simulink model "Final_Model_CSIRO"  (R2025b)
settings: Solver=ode23tb  StartTime=0.0  StopTime=50  RelTol=1e-3
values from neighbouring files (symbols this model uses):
  C_4 = 0.1670*C_b    (= 1.00487241952e-06)    [VSM_CSIRO.m]    (also in VSM.m)
  C_6 = 0.2835*C_b    (= 1.70587623314e-06)    [VSM_CSIRO.m]    (also in VSM.m)
  C_8 = 0.2275*C_b    (= 1.36891302659e-06)    [VSM_CSIRO.m]    (also in VSM.m)
  C_dc = 0.008*(n)    (= 1.6)    [VSM_CSIRO.m]    (also in VSM.m)
  C_f = n*300*10^-6    (= 0.06)    [VSM_CSIRO.m]    (also in VSM.m)
  D_p = (1/(m_p*w_b))    (= 101321.183642)    [VSM_CSIRO.m]    (also in VSM.m)
  droop_percentage = 1    [VSM_CSIRO.m]    (also in VSM.m = 5)
  i_ll = -1.15*(S_b/Vdc_n)-i_loss_dc    [VSM_CSIRO.m]    (also in VSM.m)
  i_ul = 1.15*(S_b/Vdc_n)+i_loss_dc    [VSM_CSIRO.m]    (also in VSM.m)
  J = D_p*tau_f    (= 2026.42367285)    [VSM_CSIRO.m]    (also in VSM.m)
  k_dc = eta_1/(Vdc_n*m_p)    [VSM_CSIRO.m]    (also in VSM.m)
  K_p = (1/Vdc_n)    [VSM_CSIRO.m]    (also in VSM.m)
  K_r = 1/R_dc    [VSM_CSIRO.m]    (also in VSM.m)
  Kff_i = 1    [VSM_CSIRO.m]    (also in VSM.m)
  Kff_v = 1    [VSM_CSIRO.m]    (also in VSM.m)
  Ki_i = (1/n)*1.19    (= 0.00595)    [VSM_CSIRO.m]    (also in VSM.m)
  Ki_v = (n)*1.161022    (= 232.2044)    [VSM_CSIRO.m]    (also in VSM.m)
  ki_v_ac = 4*5.2500e-04    (= 0.0021)    [VSM_CSIRO.m]    (also in VSM.m)
  Kp_i = 0.738891    [VSM_CSIRO.m]    (also in VSM.m)
  Kp_v = 0.52    [VSM_CSIRO.m]    (also in VSM.m)
  kp_v_ac = 0.001    [VSM_CSIRO.m]    (also in VSM.m)
  L1_pu = 1*0.0186/m    (= 0.000186)    [VSM_CSIRO.m]    (also in VSM.m)
  L_45 = L_lines(2)    [VSM_CSIRO.m]    (also in VSM.m)
  L_56 = L_lines(3)    [VSM_CSIRO.m]    (also in VSM.m)
  L_67 = L_lines(5)    [VSM_CSIRO.m]    (also in VSM.m)
  L_78 = L_lines(6)    [VSM_CSIRO.m]    (also in VSM.m)
  L_89 = L_lines(8)    [VSM_CSIRO.m]    (also in VSM.m)
  L_94 = L_lines(9)    [VSM_CSIRO.m]    (also in VSM.m)
  L_f = (1/n)*200*10^-6    (= 1e-06)    [VSM_CSIRO.m]    (also in VSM.m)
  n = 200    [VSM_CSIRO.m]    (also in VSM.m)
  pl = S_b*ps    (= 75000000)    [VSM_CSIRO.m]    (also in VSM.m)
  ps = base/3    (= 0.75)    [VSM_CSIRO.m]    (also in VSM.m)
  R1_pu = 1*0.00734/m    (= 7.34e-05)    [VSM_CSIRO.m]    (also in VSM.m)
  R_45 = R_lines(2)    [VSM_CSIRO.m]    (also in VSM.m)
  R_56 = R_lines(3)    [VSM_CSIRO.m]    (also in VSM.m)
  R_67 = R_lines(5)    [VSM_CSIRO.m]    (also in VSM.m)
  R_78 = R_lines(6)    [VSM_CSIRO.m]    (also in VSM.m)
  R_89 = R_lines(8)    [VSM_CSIRO.m]    (also in VSM.m)
  R_94 = R_lines(9)    [VSM_CSIRO.m]    (also in VSM.m)
  R_dc = (Vdc_n/(0.05*(S_b)/Vdc_n))    [VSM_CSIRO.m]    (also in VSM.m)
  R_f = 0.001/n    (= 5e-06)    [VSM_CSIRO.m]    (also in VSM.m)
  S_b = 100*(10^6)    (= 100000000)    [VSM_CSIRO.m]    (also in VSM.m)
  S_bt = S_b    (= 100000000)    [VSM_CSIRO.m]    (also in VSM.m)
  T_en = T_load-0.5    (= 44.5)    [VSM_CSIRO.m]    (also in VSM.m = 24.5)
  t_l = 2    [VSM_CSIRO.m]
  tau_dc = 0.05    [VSM_CSIRO.m]    (also in VSM.m)
  tau_g = 5    [VSM_CSIRO.m]    (also in VSM.m)
  V1_rms = 1000    [VSM_CSIRO.m]    (also in VSM.m)
  V2_rms = 13800    [VSM_CSIRO.m]    (also in VSM.m)
  V_m = sqrt(2/3)*V1_rms    [VSM_CSIRO.m]    (also in VSM.m)
  Vdc_n = 3*V_m    [VSM_CSIRO.m]    (also in VSM.m)
  w_b = 2*pi*f_b    (= 314.159265359)    [VSM_CSIRO.m]    (also in VSM.m)
  w_f = 2*pi*5    (= 31.4159265359)    [VSM_CSIRO.m]    (also in VSM.m)
undefined symbols (not defined in the file or in its folder): D1, Delta, DiscIntNeverNeededParam, i_dc
libraries: spsSeriesRLCBranchLib x142, spsThreePhaseVIMeasurementLib x69, slpidlib x44, spsabctodq0Lib x44, spsVoltageMeasurementLib x28, spsGroundLib x23, spsThreePhaseBreakerLib x23, spsThreePhaseParallelRLCLoadLib x21, spsdq0toabcLib x16, spsUniversalBridgeLib x16, spsPowerPositiveSequenceLib x14, spsDCVoltageSourceLib x14
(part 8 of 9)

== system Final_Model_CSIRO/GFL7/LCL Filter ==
  Cf : spsSeriesRLCBranchLib/Series RLC Branch  LConnTagsString=__new0  RConnTagsString=__new0  BranchType=RC  Resistance=200  Inductance=0.0058  SetiL0=off  InitialCurrent=0  Capacitance=50e-6  Setx0=off  InitialVoltage=0  Measurements=None
  Cf1 : spsSeriesRLCBranchLib/Series RLC Branch  LConnTagsString=__new0  RConnTagsString=__new0  BranchType=RC  Resistance=200  Inductance=0.0058  SetiL0=off  InitialCurrent=0  Capacitance=50e-6  Setx0=off  InitialVoltage=0  Measurements=None
  Cf2 : spsSeriesRLCBranchLib/Series RLC Branch  LConnTagsString=__new0  RConnTagsString=__new0  BranchType=RC  Resistance=200  Inductance=0.0058  SetiL0=off  InitialCurrent=0  Capacitance=50e-6  Setx0=off  InitialVoltage=0  Measurements=None
  Ground : spsGroundLib/Ground  LConnTagsString=a
  Lg : spsSeriesRLCBranchLib/Series RLC Branch  LConnTagsString=__new0  RConnTagsString=__new0  BranchType=L  Resistance=0.2  Inductance=5e-6  SetiL0=off  InitialCurrent=0  Capacitance=1e-6  Setx0=off  InitialVoltage=0  Measurements=None
  Linv : spsSeriesRLCBranchLib/Series RLC Branch  LConnTagsString=__new0  RConnTagsString=__new0  BranchType=RL  Resistance=1e-3  Inductance=0.003e-3  SetiL0=off  InitialCurrent=0  Capacitance=1e-6  Setx0=off  InitialVoltage=0  Measurements=None
  Series RLC Branch1 : spsSeriesRLCBranchLib/Series RLC Branch  LConnTagsString=__new0  RConnTagsString=__new0  BranchType=RL  Resistance=1e-3  Inductance=0.003e-3  SetiL0=off  InitialCurrent=0  Capacitance=1e-6  Setx0=off  InitialVoltage=0  Measurements=None
  Series RLC Branch2 : spsSeriesRLCBranchLib/Series RLC Branch  LConnTagsString=__new0  RConnTagsString=__new0  BranchType=RL  Resistance=1e-3  Inductance=0.003e-3  SetiL0=off  InitialCurrent=0  Capacitance=1e-6  Setx0=off  InitialVoltage=0  Measurements=None
  Series RLC Branch3 : spsSeriesRLCBranchLib/Series RLC Branch  LConnTagsString=__new0  RConnTagsString=__new0  BranchType=L  Resistance=0.2  Inductance=5e-6  SetiL0=off  InitialCurrent=0  Capacitance=1e-6  Setx0=off  InitialVoltage=0  Measurements=None
  Series RLC Branch4 : spsSeriesRLCBranchLib/Series RLC Branch  LConnTagsString=__new0  RConnTagsString=__new0  BranchType=L  Resistance=0.2  Inductance=5e-6  SetiL0=off  InitialCurrent=0  Capacitance=1e-6  Setx0=off  InitialVoltage=0  Measurements=None
  Three-Phase V-I Measurement : spsThreePhaseVIMeasurementLib/Three-Phase V-I Measurement  VoltageMeasurement=phase-to-phase  SetLabelV=on  LabelV=Vabc_B2_8  Vpu=off  VpuLL=off  CurrentMeasurement=no  SetLabelI=off  LabelI=Iabc  Ipu=off  Pbase=100e6  Vbase=500e3  OutputType=Complex  PhasorSimulation=off  PSBequivalent=0
  A : PMIOPort  Side=Left
  a : PMIOPort  Port=2  Side=Right
  B : PMIOPort  Port=3  Side=Left
  b : PMIOPort  Port=4  Side=Right
  C : PMIOPort  Port=5  Side=Left
  c : PMIOPort  Port=6  Side=Right
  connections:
  A/RConn1 -- Linv/LConn1
  B/RConn1 -- Series RLC Branch1/LConn1
  C/RConn1 -- Series RLC Branch2/LConn1
  Lg/LConn1 -- Three-Phase V-I Measurement/LConn1 -- Linv/RConn1
  Series RLC Branch4/LConn1 -- Three-Phase V-I Measurement/LConn3 -- Series RLC Branch2/RConn1
  Series RLC Branch3/LConn1 -- Three-Phase V-I Measurement/LConn2 -- Series RLC Branch1/RConn1
  Cf1/LConn1 -- Ground/LConn1 -- Cf/LConn1 -- Cf2/LConn1
  Cf/RConn1 -- Three-Phase V-I Measurement/RConn1
  Cf1/RConn1 -- Three-Phase V-I Measurement/RConn2
  Cf2/RConn1 -- Three-Phase V-I Measurement/RConn3
  Lg/RConn1 -- a/RConn1
  Series RLC Branch3/RConn1 -- b/RConn1
  Series RLC Branch4/RConn1 -- c/RConn1

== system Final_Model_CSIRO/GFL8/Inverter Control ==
  note: PLL
  Vabc_B3 : Inport
  Iabc_B3 : Inport  Port=2
  Idref : Inport  Port=3
  Iqref : Inport  Port=4
  Clock : Clock
  Constant : Constant  Value=0  SampleTime=-1
  Constant1 : Constant  Value=0  SampleTime=-1
  Constant3 : Constant  Value=314.159  SampleTime=-1
  Constant4 : Constant  Value=0
  Demux : Demux  Outputs=3
  Demux1 : Demux  Outputs=3
  Discrete-Time Integrator : DiscreteIntegrator  SampleTime=-1  ICPrevOutput=DiscIntNeverNeededParam  ICPrevScaledInput=DiscIntNeverNeededParam
  Gain : Gain  Gain=2/1800
  Memory : Memory
  Mux : Mux  Inputs=3
  PID Controller : slpidlib/PID Controller  Controller=PI  Form=Parallel  TimeDomain=Discrete-time  UseExternalTs=off  SampleTime=-1  IntegratorMethod=Forward Euler  FilterMethod=Forward Euler  ControllerParametersSource=internal  P=0.02  I=50  UseKiTs=off  D=0  UseExternalDerivativeSource=off  N=100  UseFilter=on  TunerSelectOption=Transfer Function Based (PID Tuner App)  InitialConditionSource=internal  InitialConditionForIntegrator=0  InitialConditionForFilter=0  DifferentiatorICPrevScaledInput=0  ExternalReset=none  TrackingMode=off  Kt=1  LimitOutput=off  SatLimitsSource=internal  UpperSaturationLimit=inf  LowerSaturationLimit=-inf  LinearizeAsGain=on  AntiWindupMode=none  Kb=1  LimitIntegrator=off  UpperIntegratorSaturationLimit=inf  LowerIntegratorSaturationLimit=-inf  POutMin=[]  POutMax=[]  IOutMin=[]  IOutMax=[]  DOutMin=[]  DOutMax=[]  NOutMin=[]  NOutMax=[]  SumOutMin=[]  SumOutMax=[]  SaturationOutMin=[]  SaturationOutMax=[]  PParamMin=[]  PParamMax=[]  IParamMin=[]  IParamMax=[]  DParamMin=[]  DParamMax=[]  NParamMin=[]  NParamMax=[]  KbParamMin=[]  KbParamMax=[]  KtParamMin=[]  KtParamMax=[]  KbOutMin=[]  KbOutMax=[]  KtOutMin=[]  KtOutMax=[]  IntegratorOutMin=[]  IntegratorOutMax=[]  FilterOutMin=[]  FilterOutMax=[]  SumI1OutMin=[]  SumI1OutMax=[]  SumI2OutMin=[]  SumI2OutMax=[]  SumI3OutMin=[]  SumI3OutMax=[]  SumI4OutMin=[]  SumI4OutMax=[]  SumDOutMin=[]  SumDOutMax=[]  DifferentiatorOutMin=[]  DifferentiatorOutMax=[]  FilterDiffOutCoefMin=[]  FilterDiffOutCoefMax=[]  ReciprocalOutMin=[]  ReciprocalOutMax=[]  SumDenOutMin=[]  SumDenOutMax=[]  SumNumOutMin=[]  SumNumOutMax=[]  DivideOutMin=[]  DivideOutMax=[]  UdiffTsProdOutMin=[]  UdiffTsProdOutMax=[]  NTsProdOutMin=[]  NTsProdOutMax=[]  UintegralTsProdOutMin=[]  UintegralTsProdOutMax=[]  UngainTsProdOutMin=[]  UngainTsProdOutMax=[]  ClampingZeroOutDataTypeStr=Inherit: Inherit via back propagation  ClampingZeroOutMin=[]  ClampingZeroOutMax=[]  FilterDenConstantOutDataTypeStr=Inherit: Inherit via back propagation  FilterDenConstantOutMin=[]  FilterDenConstantOutMax=[]  PCopyOutDataTypeStr=Inherit: Inherit via back propagation  PCopyOutMin=[]  PCopyOutMax=[]  NCopyOutDataTypeStr=Inherit: Inherit via back propagation  NCopyOutMin=[]  NCopyOutMax=[]  IntegratorContinuousStateAttributes=''  IntegratorStateMustResolveToSignalObject=off  IntegratorRTWStateStorageClass=Auto  FilterContinuousStateAttributes=''  FilterStateMustResolveToSignalObject=off  FilterRTWStateStorageClass=Auto  ParallelPVariant=InternalParameters  IdealPVariant=Disabled  IVariant=InternalParameters  DVariant=Disabled  IntegratorVariant=Discrete  SatVariant=Disabled  AWVariant=Passthrough  PCopyVariant=Disabled  TRVariant=Disabled  FdbkBlocksVariant=Forward  IdealPFdbkVariant=Disabled  SatFdbkVariant=Disabled  DerivativeFilterVariant=Disabled  NVariant=Disabled  NCopyVariant=Disabled_SignalSpec  FilterICVariant=Disabled  IntegratorICVariant=InternalICs  ExternalResetVariant=Disabled  TRSumVariant=Passthrough  SumFdbkVariant=Disabled  SumVariant=Sum_PI  TsampFilterVariant=InternalTs  TsampNgainVariant=Passthrough  TsampIntegralVariant=Disabled_SignalSpec  ExternalSaturationOutDataTypeStr=Inherit: Same as second input  DerivativeSourceVariant=Disabled  PreIntVariant=InternalPreInt
  PID Controller1 : slpidlib/PID Controller  Controller=PI  Form=Parallel  TimeDomain=Discrete-time  UseExternalTs=off  SampleTime=-1  IntegratorMethod=Forward Euler  FilterMethod=Forward Euler  ControllerParametersSource=internal  P=0.1  I=10000/200  UseKiTs=off  D=0  UseExternalDerivativeSource=off  N=100  UseFilter=on  TunerSelectOption=Transfer Function Based (PID Tuner App)  InitialConditionSource=internal  InitialConditionForIntegrator=0  InitialConditionForFilter=0  DifferentiatorICPrevScaledInput=0  ExternalReset=none  TrackingMode=off  Kt=1  LimitOutput=on  SatLimitsSource=internal  UpperSaturationLimit=20e3  LowerSaturationLimit=-20e3  LinearizeAsGain=on  AntiWindupMode=none  Kb=1  LimitIntegrator=off  UpperIntegratorSaturationLimit=inf  LowerIntegratorSaturationLimit=-inf  POutMin=[]  POutMax=[]  IOutMin=[]  IOutMax=[]  DOutMin=[]  DOutMax=[]  NOutMin=[]  NOutMax=[]  SumOutMin=[]  SumOutMax=[]  SaturationOutMin=[]  SaturationOutMax=[]  PParamMin=[]  PParamMax=[]  IParamMin=[]  IParamMax=[]  DParamMin=[]  DParamMax=[]  NParamMin=[]  NParamMax=[]  KbParamMin=[]  KbParamMax=[]  KtParamMin=[]  KtParamMax=[]  KbOutMin=[]  KbOutMax=[]  KtOutMin=[]  KtOutMax=[]  IntegratorOutMin=[]  IntegratorOutMax=[]  FilterOutMin=[]  FilterOutMax=[]  SumI1OutMin=[]  SumI1OutMax=[]  SumI2OutMin=[]  SumI2OutMax=[]  SumI3OutMin=[]  SumI3OutMax=[]  SumI4OutMin=[]  SumI4OutMax=[]  SumDOutMin=[]  SumDOutMax=[]  DifferentiatorOutMin=[]  DifferentiatorOutMax=[]  FilterDiffOutCoefMin=[]  FilterDiffOutCoefMax=[]  ReciprocalOutMin=[]  ReciprocalOutMax=[]  SumDenOutMin=[]  SumDenOutMax=[]  SumNumOutMin=[]  SumNumOutMax=[]  DivideOutMin=[]  DivideOutMax=[]  UdiffTsProdOutMin=[]  UdiffTsProdOutMax=[]  NTsProdOutMin=[]  NTsProdOutMax=[]  UintegralTsProdOutMin=[]  UintegralTsProdOutMax=[]  UngainTsProdOutMin=[]  UngainTsProdOutMax=[]  ClampingZeroOutDataTypeStr=Inherit: Inherit via back propagation  ClampingZeroOutMin=[]  ClampingZeroOutMax=[]  FilterDenConstantOutDataTypeStr=Inherit: Inherit via back propagation  FilterDenConstantOutMin=[]  FilterDenConstantOutMax=[]  PCopyOutDataTypeStr=Inherit: Inherit via back propagation  PCopyOutMin=[]  PCopyOutMax=[]  NCopyOutDataTypeStr=Inherit: Inherit via back propagation  NCopyOutMin=[]  NCopyOutMax=[]  IntegratorContinuousStateAttributes=''  IntegratorStateMustResolveToSignalObject=off  IntegratorRTWStateStorageClass=Auto  FilterContinuousStateAttributes=''  FilterStateMustResolveToSignalObject=off  FilterRTWStateStorageClass=Auto  ParallelPVariant=InternalParameters  IdealPVariant=Disabled  IVariant=InternalParameters  DVariant=Disabled  IntegratorVariant=Discrete  SatVariant=Enabled  AWVariant=Passthrough  PCopyVariant=Disabled  TRVariant=Disabled  FdbkBlocksVariant=Forward  IdealPFdbkVariant=Disabled  SatFdbkVariant=Disabled  DerivativeFilterVariant=Disabled  NVariant=Disabled  NCopyVariant=Disabled_SignalSpec  FilterICVariant=Disabled  IntegratorICVariant=InternalICs  ExternalResetVariant=Disabled  TRSumVariant=Passthrough  SumFdbkVariant=Disabled  SumVariant=Sum_PI  TsampFilterVariant=InternalTs  TsampNgainVariant=Passthrough  TsampIntegralVariant=Disabled_SignalSpec  ExternalSaturationOutDataTypeStr=Inherit: Same as second input  DerivativeSourceVariant=Disabled  PreIntVariant=InternalPreInt
  PID Controller2 : slpidlib/PID Controller  Controller=PI  Form=Parallel  TimeDomain=Discrete-time  UseExternalTs=off  SampleTime=-1  IntegratorMethod=Forward Euler  FilterMethod=Forward Euler  ControllerParametersSource=internal  P=0.1  I=1000/2  UseKiTs=off  D=0  UseExternalDerivativeSource=off  N=100  UseFilter=on  TunerSelectOption=Transfer Function Based (PID Tuner App)  InitialConditionSource=internal  InitialConditionForIntegrator=0  InitialConditionForFilter=0  DifferentiatorICPrevScaledInput=0  ExternalReset=none  TrackingMode=off  Kt=1  LimitOutput=on  SatLimitsSource=internal  UpperSaturationLimit=20e3  LowerSaturationLimit=-20e3  LinearizeAsGain=on  AntiWindupMode=none  Kb=1  LimitIntegrator=off  UpperIntegratorSaturationLimit=inf  LowerIntegratorSaturationLimit=-inf  POutMin=[]  POutMax=[]  IOutMin=[]  IOutMax=[]  DOutMin=[]  DOutMax=[]  NOutMin=[]  NOutMax=[]  SumOutMin=[]  SumOutMax=[]  SaturationOutMin=[]  SaturationOutMax=[]  PParamMin=[]  PParamMax=[]  IParamMin=[]  IParamMax=[]  DParamMin=[]  DParamMax=[]  NParamMin=[]  NParamMax=[]  KbParamMin=[]  KbParamMax=[]  KtParamMin=[]  KtParamMax=[]  KbOutMin=[]  KbOutMax=[]  KtOutMin=[]  KtOutMax=[]  IntegratorOutMin=[]  IntegratorOutMax=[]  FilterOutMin=[]  FilterOutMax=[]  SumI1OutMin=[]  SumI1OutMax=[]  SumI2OutMin=[]  SumI2OutMax=[]  SumI3OutMin=[]  SumI3OutMax=[]  SumI4OutMin=[]  SumI4OutMax=[]  SumDOutMin=[]  SumDOutMax=[]  DifferentiatorOutMin=[]  DifferentiatorOutMax=[]  FilterDiffOutCoefMin=[]  FilterDiffOutCoefMax=[]  ReciprocalOutMin=[]  ReciprocalOutMax=[]  SumDenOutMin=[]  SumDenOutMax=[]  SumNumOutMin=[]  SumNumOutMax=[]  DivideOutMin=[]  DivideOutMax=[]  UdiffTsProdOutMin=[]  UdiffTsProdOutMax=[]  NTsProdOutMin=[]  NTsProdOutMax=[]  UintegralTsProdOutMin=[]  UintegralTsProdOutMax=[]  UngainTsProdOutMin=[]  UngainTsProdOutMax=[]  ClampingZeroOutDataTypeStr=Inherit: Inherit via back propagation  ClampingZeroOutMin=[]  ClampingZeroOutMax=[]  FilterDenConstantOutDataTypeStr=Inherit: Inherit via back propagation  FilterDenConstantOutMin=[]  FilterDenConstantOutMax=[]  PCopyOutDataTypeStr=Inherit: Inherit via back propagation  PCopyOutMin=[]  PCopyOutMax=[]  NCopyOutDataTypeStr=Inherit: Inherit via back propagation  NCopyOutMin=[]  NCopyOutMax=[]  IntegratorContinuousStateAttributes=''  IntegratorStateMustResolveToSignalObject=off  IntegratorRTWStateStorageClass=Auto  FilterContinuousStateAttributes=''  FilterStateMustResolveToSignalObject=off  FilterRTWStateStorageClass=Auto  ParallelPVariant=InternalParameters  IdealPVariant=Disabled  IVariant=InternalParameters  DVariant=Disabled  IntegratorVariant=Discrete  SatVariant=Enabled  AWVariant=Passthrough  PCopyVariant=Disabled  TRVariant=Disabled  FdbkBlocksVariant=Forward  IdealPFdbkVariant=Disabled  SatFdbkVariant=Disabled  DerivativeFilterVariant=Disabled  NVariant=Disabled  NCopyVariant=Disabled_SignalSpec  FilterICVariant=Disabled  IntegratorICVariant=InternalICs  ExternalResetVariant=Disabled  TRSumVariant=Passthrough  SumFdbkVariant=Disabled  SumVariant=Sum_PI  TsampFilterVariant=InternalTs  TsampNgainVariant=Passthrough  TsampIntegralVariant=Disabled_SignalSpec  ExternalSaturationOutDataTypeStr=Inherit: Same as second input  DerivativeSourceVariant=Disabled  PreIntVariant=InternalPreInt
  Saturation : Saturate  UpperLimit=1  LowerLimit=-1
  Scope : Scope  NumInputPorts=2
  Scope4 : Scope  NumInputPorts=2
  Sum : Sum  Inputs=|-+
  Sum1 : Sum  Inputs=|+-
  Sum2 : Sum  Inputs=|+-
  Sum3 : Sum  Inputs=|+-
  Sum{4..6,8} (4 alike) : Sum  Inputs=|++
  Switch : Switch  Criteria=u2 > Threshold  Threshold=10
  Terminator : Terminator
  Terminator1 : Terminator
  abc to dq0 : spsabctodq0Lib/abc to dq0  Alignment=90 degrees behind phase A axis
  abc to dq1 : spsabctodq0Lib/abc to dq0  Alignment=90 degrees behind phase A axis
  dq0 to abc : spsdq0toabcLib/dq0 to abc  Alignment=90 degrees behind phase A axis
  wL : Gain  Gain=0.314*0.003
  wL1 : Gain  Gain=0.314*0.003
  Pulses : Outport
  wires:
  abc to dq0/1 -> Demux/1
  Demux/3 -> Terminator/1
  Demux1/3 -> Terminator1/1
  abc to dq1/1 -> Demux1/1
  Iabc_B3/1 -> abc to dq1/1
  Constant/1 -> Sum/1
  Demux/2 -> [Vq]  "Vq"
  Sum/1 -> PID Controller/1
  PID Controller/1 -> Sum8/1
  [wt] -> abc to dq1/2, abc to dq0/2
  Demux1/1 -> [Id]  "Id"
  Demux1/2 -> [Iq]  "Iq"
  [Id] -> Scope/2, Sum1/2
  Iqref/1 -> Scope4/1, Sum2/1
  [Iq] -> Sum2/2, Scope4/2
  Sum1/1 -> PID Controller1/1
  Sum2/1 -> PID Controller2/1
  PID Controller1/1 -> Sum3/1
  PID Controller2/1 -> Sum4/1
  wL1/1 -> Sum4/2
  wL/1 -> Sum3/2
  Sum3/1 -> Sum5/1
  [Vd] -> Sum5/2
  Sum4/1 -> Sum6/1
  [Vq] -> Sum6/2
  Mux/1 -> dq0 to abc/1
  Sum5/1 -> Mux/1  "ud"
  Sum6/1 -> Mux/2  "uq"
  Constant1/1 -> Mux/3
  dq0 to abc/1 -> Gain/1
  Vabc_B3/1 -> abc to dq0/1
  Idref/1 -> Scope/1, Sum1/1
  [Id] -> wL1/1
  [Iq] -> wL/1
  Demux/1 -> [Vd]  "Vd"
  Gain/1 -> Saturation/1
  Memory/1 -> Pulses/1
  Discrete-Time Integrator/1 -> [wt]
  Saturation/1 -> Memory/1
  Constant3/1 -> Sum8/2
  Switch/1 -> Sum/2
  Constant4/1 -> Switch/3
  Clock/1 -> Switch/2
  [Vq] -> Switch/1
  [wt] -> dq0 to abc/2
  Sum8/1 -> Discrete-Time Integrator/1

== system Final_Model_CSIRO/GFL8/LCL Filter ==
  Cf : spsSeriesRLCBranchLib/Series RLC Branch  LConnTagsString=__new0  RConnTagsString=__new0  BranchType=RC  Resistance=200  Inductance=0.0058  SetiL0=off  InitialCurrent=0  Capacitance=50e-6  Setx0=off  InitialVoltage=0  Measurements=None
  Cf1 : spsSeriesRLCBranchLib/Series RLC Branch  LConnTagsString=__new0  RConnTagsString=__new0  BranchType=RC  Resistance=200  Inductance=0.0058  SetiL0=off  InitialCurrent=0  Capacitance=50e-6  Setx0=off  InitialVoltage=0  Measurements=None
  Cf2 : spsSeriesRLCBranchLib/Series RLC Branch  LConnTagsString=__new0  RConnTagsString=__new0  BranchType=RC  Resistance=200  Inductance=0.0058  SetiL0=off  InitialCurrent=0  Capacitance=50e-6  Setx0=off  InitialVoltage=0  Measurements=None
  Ground : spsGroundLib/Ground  LConnTagsString=a
  Lg : spsSeriesRLCBranchLib/Series RLC Branch  LConnTagsString=__new0  RConnTagsString=__new0  BranchType=L  Resistance=0.2  Inductance=5e-6  SetiL0=off  InitialCurrent=0  Capacitance=1e-6  Setx0=off  InitialVoltage=0  Measurements=None
  Linv : spsSeriesRLCBranchLib/Series RLC Branch  LConnTagsString=__new0  RConnTagsString=__new0  BranchType=RL  Resistance=1e-3  Inductance=0.003e-3  SetiL0=off  InitialCurrent=0  Capacitance=1e-6  Setx0=off  InitialVoltage=0  Measurements=None
  Series RLC Branch1 : spsSeriesRLCBranchLib/Series RLC Branch  LConnTagsString=__new0  RConnTagsString=__new0  BranchType=RL  Resistance=1e-3  Inductance=0.003e-3  SetiL0=off  InitialCurrent=0  Capacitance=1e-6  Setx0=off  InitialVoltage=0  Measurements=None
  Series RLC Branch2 : spsSeriesRLCBranchLib/Series RLC Branch  LConnTagsString=__new0  RConnTagsString=__new0  BranchType=RL  Resistance=1e-3  Inductance=0.003e-3  SetiL0=off  InitialCurrent=0  Capacitance=1e-6  Setx0=off  InitialVoltage=0  Measurements=None
  Series RLC Branch3 : spsSeriesRLCBranchLib/Series RLC Branch  LConnTagsString=__new0  RConnTagsString=__new0  BranchType=L  Resistance=0.2  Inductance=5e-6  SetiL0=off  InitialCurrent=0  Capacitance=1e-6  Setx0=off  InitialVoltage=0  Measurements=None
  Series RLC Branch4 : spsSeriesRLCBranchLib/Series RLC Branch  LConnTagsString=__new0  RConnTagsString=__new0  BranchType=L  Resistance=0.2  Inductance=5e-6  SetiL0=off  InitialCurrent=0  Capacitance=1e-6  Setx0=off  InitialVoltage=0  Measurements=None
  Three-Phase V-I Measurement : spsThreePhaseVIMeasurementLib/Three-Phase V-I Measurement  VoltageMeasurement=phase-to-phase  SetLabelV=on  LabelV=Vabc_B2_9  Vpu=off  VpuLL=off  CurrentMeasurement=no  SetLabelI=off  LabelI=Iabc  Ipu=off  Pbase=100e6  Vbase=500e3  OutputType=Complex  PhasorSimulation=off  PSBequivalent=0
  A : PMIOPort  Side=Left
  a : PMIOPort  Port=2  Side=Right
  B : PMIOPort  Port=3  Side=Left
  b : PMIOPort  Port=4  Side=Right
  C : PMIOPort  Port=5  Side=Left
  c : PMIOPort  Port=6  Side=Right
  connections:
  A/RConn1 -- Linv/LConn1
  B/RConn1 -- Series RLC Branch1/LConn1
  C/RConn1 -- Series RLC Branch2/LConn1
  Lg/LConn1 -- Three-Phase V-I Measurement/LConn1 -- Linv/RConn1
  Series RLC Branch4/LConn1 -- Three-Phase V-I Measurement/LConn3 -- Series RLC Branch2/RConn1
  Series RLC Branch3/LConn1 -- Three-Phase V-I Measurement/LConn2 -- Series RLC Branch1/RConn1
  Cf1/LConn1 -- Ground/LConn1 -- Cf/LConn1 -- Cf2/LConn1
  Cf/RConn1 -- Three-Phase V-I Measurement/RConn1
  Cf1/RConn1 -- Three-Phase V-I Measurement/RConn2
  Cf2/RConn1 -- Three-Phase V-I Measurement/RConn3
  Lg/RConn1 -- a/RConn1
  Series RLC Branch3/RConn1 -- b/RConn1
  Series RLC Branch4/RConn1 -- c/RConn1

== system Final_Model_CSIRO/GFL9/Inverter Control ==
  note: PLL
  Vabc_B3 : Inport
  Iabc_B3 : Inport  Port=2
  Idref : Inport  Port=3
  Iqref : Inport  Port=4
  Clock : Clock
  Constant : Constant  Value=0  SampleTime=-1
  Constant1 : Constant  Value=0  SampleTime=-1
  Constant3 : Constant  Value=314.159  SampleTime=-1
  Constant4 : Constant  Value=0
  Demux : Demux  Outputs=3
  Demux1 : Demux  Outputs=3
  Discrete-Time Integrator : DiscreteIntegrator  SampleTime=-1  ICPrevOutput=DiscIntNeverNeededParam  ICPrevScaledInput=DiscIntNeverNeededParam
  Gain : Gain  Gain=2/1800
  Memory : Memory
  Mux : Mux  Inputs=3
  PID Controller : slpidlib/PID Controller  Controller=PI  Form=Parallel  TimeDomain=Discrete-time  UseExternalTs=off  SampleTime=-1  IntegratorMethod=Forward Euler  FilterMethod=Forward Euler  ControllerParametersSource=internal  P=0.02  I=50  UseKiTs=off  D=0  UseExternalDerivativeSource=off  N=100  UseFilter=on  TunerSelectOption=Transfer Function Based (PID Tuner App)  InitialConditionSource=internal  InitialConditionForIntegrator=0  InitialConditionForFilter=0  DifferentiatorICPrevScaledInput=0  ExternalReset=none  TrackingMode=off  Kt=1  LimitOutput=off  SatLimitsSource=internal  UpperSaturationLimit=inf  LowerSaturationLimit=-inf  LinearizeAsGain=on  AntiWindupMode=none  Kb=1  LimitIntegrator=off  UpperIntegratorSaturationLimit=inf  LowerIntegratorSaturationLimit=-inf  POutMin=[]  POutMax=[]  IOutMin=[]  IOutMax=[]  DOutMin=[]  DOutMax=[]  NOutMin=[]  NOutMax=[]  SumOutMin=[]  SumOutMax=[]  SaturationOutMin=[]  SaturationOutMax=[]  PParamMin=[]  PParamMax=[]  IParamMin=[]  IParamMax=[]  DParamMin=[]  DParamMax=[]  NParamMin=[]  NParamMax=[]  KbParamMin=[]  KbParamMax=[]  KtParamMin=[]  KtParamMax=[]  KbOutMin=[]  KbOutMax=[]  KtOutMin=[]  KtOutMax=[]  IntegratorOutMin=[]  IntegratorOutMax=[]  FilterOutMin=[]  FilterOutMax=[]  SumI1OutMin=[]  SumI1OutMax=[]  SumI2OutMin=[]  SumI2OutMax=[]  SumI3OutMin=[]  SumI3OutMax=[]  SumI4OutMin=[]  SumI4OutMax=[]  SumDOutMin=[]  SumDOutMax=[]  DifferentiatorOutMin=[]  DifferentiatorOutMax=[]  FilterDiffOutCoefMin=[]  FilterDiffOutCoefMax=[]  ReciprocalOutMin=[]  ReciprocalOutMax=[]  SumDenOutMin=[]  SumDenOutMax=[]  SumNumOutMin=[]  SumNumOutMax=[]  DivideOutMin=[]  DivideOutMax=[]  UdiffTsProdOutMin=[]  UdiffTsProdOutMax=[]  NTsProdOutMin=[]  NTsProdOutMax=[]  UintegralTsProdOutMin=[]  UintegralTsProdOutMax=[]  UngainTsProdOutMin=[]  UngainTsProdOutMax=[]  ClampingZeroOutDataTypeStr=Inherit: Inherit via back propagation  ClampingZeroOutMin=[]  ClampingZeroOutMax=[]  FilterDenConstantOutDataTypeStr=Inherit: Inherit via back propagation  FilterDenConstantOutMin=[]  FilterDenConstantOutMax=[]  PCopyOutDataTypeStr=Inherit: Inherit via back propagation  PCopyOutMin=[]  PCopyOutMax=[]  NCopyOutDataTypeStr=Inherit: Inherit via back propagation  NCopyOutMin=[]  NCopyOutMax=[]  IntegratorContinuousStateAttributes=''  IntegratorStateMustResolveToSignalObject=off  IntegratorRTWStateStorageClass=Auto  FilterContinuousStateAttributes=''  FilterStateMustResolveToSignalObject=off  FilterRTWStateStorageClass=Auto  ParallelPVariant=InternalParameters  IdealPVariant=Disabled  IVariant=InternalParameters  DVariant=Disabled  IntegratorVariant=Discrete  SatVariant=Disabled  AWVariant=Passthrough  PCopyVariant=Disabled  TRVariant=Disabled  FdbkBlocksVariant=Forward  IdealPFdbkVariant=Disabled  SatFdbkVariant=Disabled  DerivativeFilterVariant=Disabled  NVariant=Disabled  NCopyVariant=Disabled_SignalSpec  FilterICVariant=Disabled  IntegratorICVariant=InternalICs  ExternalResetVariant=Disabled  TRSumVariant=Passthrough  SumFdbkVariant=Disabled  SumVariant=Sum_PI  TsampFilterVariant=InternalTs  TsampNgainVariant=Passthrough  TsampIntegralVariant=Disabled_SignalSpec  ExternalSaturationOutDataTypeStr=Inherit: Same as second input  DerivativeSourceVariant=Disabled  PreIntVariant=InternalPreInt
  PID Controller1 : slpidlib/PID Controller  Controller=PI  Form=Parallel  TimeDomain=Discrete-time  UseExternalTs=off  SampleTime=-1  IntegratorMethod=Forward Euler  FilterMethod=Forward Euler  ControllerParametersSource=internal  P=0.1  I=10000/200  UseKiTs=off  D=0  UseExternalDerivativeSource=off  N=100  UseFilter=on  TunerSelectOption=Transfer Function Based (PID Tuner App)  InitialConditionSource=internal  InitialConditionForIntegrator=0  InitialConditionForFilter=0  DifferentiatorICPrevScaledInput=0  ExternalReset=none  TrackingMode=off  Kt=1  LimitOutput=on  SatLimitsSource=internal  UpperSaturationLimit=20e3  LowerSaturationLimit=-20e3  LinearizeAsGain=on  AntiWindupMode=none  Kb=1  LimitIntegrator=off  UpperIntegratorSaturationLimit=inf  LowerIntegratorSaturationLimit=-inf  POutMin=[]  POutMax=[]  IOutMin=[]  IOutMax=[]  DOutMin=[]  DOutMax=[]  NOutMin=[]  NOutMax=[]  SumOutMin=[]  SumOutMax=[]  SaturationOutMin=[]  SaturationOutMax=[]  PParamMin=[]  PParamMax=[]  IParamMin=[]  IParamMax=[]  DParamMin=[]  DParamMax=[]  NParamMin=[]  NParamMax=[]  KbParamMin=[]  KbParamMax=[]  KtParamMin=[]  KtParamMax=[]  KbOutMin=[]  KbOutMax=[]  KtOutMin=[]  KtOutMax=[]  IntegratorOutMin=[]  IntegratorOutMax=[]  FilterOutMin=[]  FilterOutMax=[]  SumI1OutMin=[]  SumI1OutMax=[]  SumI2OutMin=[]  SumI2OutMax=[]  SumI3OutMin=[]  SumI3OutMax=[]  SumI4OutMin=[]  SumI4OutMax=[]  SumDOutMin=[]  SumDOutMax=[]  DifferentiatorOutMin=[]  DifferentiatorOutMax=[]  FilterDiffOutCoefMin=[]  FilterDiffOutCoefMax=[]  ReciprocalOutMin=[]  ReciprocalOutMax=[]  SumDenOutMin=[]  SumDenOutMax=[]  SumNumOutMin=[]  SumNumOutMax=[]  DivideOutMin=[]  DivideOutMax=[]  UdiffTsProdOutMin=[]  UdiffTsProdOutMax=[]  NTsProdOutMin=[]  NTsProdOutMax=[]  UintegralTsProdOutMin=[]  UintegralTsProdOutMax=[]  UngainTsProdOutMin=[]  UngainTsProdOutMax=[]  ClampingZeroOutDataTypeStr=Inherit: Inherit via back propagation  ClampingZeroOutMin=[]  ClampingZeroOutMax=[]  FilterDenConstantOutDataTypeStr=Inherit: Inherit via back propagation  FilterDenConstantOutMin=[]  FilterDenConstantOutMax=[]  PCopyOutDataTypeStr=Inherit: Inherit via back propagation  PCopyOutMin=[]  PCopyOutMax=[]  NCopyOutDataTypeStr=Inherit: Inherit via back propagation  NCopyOutMin=[]  NCopyOutMax=[]  IntegratorContinuousStateAttributes=''  IntegratorStateMustResolveToSignalObject=off  IntegratorRTWStateStorageClass=Auto  FilterContinuousStateAttributes=''  FilterStateMustResolveToSignalObject=off  FilterRTWStateStorageClass=Auto  ParallelPVariant=InternalParameters  IdealPVariant=Disabled  IVariant=InternalParameters  DVariant=Disabled  IntegratorVariant=Discrete  SatVariant=Enabled  AWVariant=Passthrough  PCopyVariant=Disabled  TRVariant=Disabled  FdbkBlocksVariant=Forward  IdealPFdbkVariant=Disabled  SatFdbkVariant=Disabled  DerivativeFilterVariant=Disabled  NVariant=Disabled  NCopyVariant=Disabled_SignalSpec  FilterICVariant=Disabled  IntegratorICVariant=InternalICs  ExternalResetVariant=Disabled  TRSumVariant=Passthrough  SumFdbkVariant=Disabled  SumVariant=Sum_PI  TsampFilterVariant=InternalTs  TsampNgainVariant=Passthrough  TsampIntegralVariant=Disabled_SignalSpec  ExternalSaturationOutDataTypeStr=Inherit: Same as second input  DerivativeSourceVariant=Disabled  PreIntVariant=InternalPreInt
  PID Controller2 : slpidlib/PID Controller  Controller=PI  Form=Parallel  TimeDomain=Discrete-time  UseExternalTs=off  SampleTime=-1  IntegratorMethod=Forward Euler  FilterMethod=Forward Euler  ControllerParametersSource=internal  P=0.1  I=1000/2  UseKiTs=off  D=0  UseExternalDerivativeSource=off  N=100  UseFilter=on  TunerSelectOption=Transfer Function Based (PID Tuner App)  InitialConditionSource=internal  InitialConditionForIntegrator=0  InitialConditionForFilter=0  DifferentiatorICPrevScaledInput=0  ExternalReset=none  TrackingMode=off  Kt=1  LimitOutput=on  SatLimitsSource=internal  UpperSaturationLimit=20e3  LowerSaturationLimit=-20e3  LinearizeAsGain=on  AntiWindupMode=none  Kb=1  LimitIntegrator=off  UpperIntegratorSaturationLimit=inf  LowerIntegratorSaturationLimit=-inf  POutMin=[]  POutMax=[]  IOutMin=[]  IOutMax=[]  DOutMin=[]  DOutMax=[]  NOutMin=[]  NOutMax=[]  SumOutMin=[]  SumOutMax=[]  SaturationOutMin=[]  SaturationOutMax=[]  PParamMin=[]  PParamMax=[]  IParamMin=[]  IParamMax=[]  DParamMin=[]  DParamMax=[]  NParamMin=[]  NParamMax=[]  KbParamMin=[]  KbParamMax=[]  KtParamMin=[]  KtParamMax=[]  KbOutMin=[]  KbOutMax=[]  KtOutMin=[]  KtOutMax=[]  IntegratorOutMin=[]  IntegratorOutMax=[]  FilterOutMin=[]  FilterOutMax=[]  SumI1OutMin=[]  SumI1OutMax=[]  SumI2OutMin=[]  SumI2OutMax=[]  SumI3OutMin=[]  SumI3OutMax=[]  SumI4OutMin=[]  SumI4OutMax=[]  SumDOutMin=[]  SumDOutMax=[]  DifferentiatorOutMin=[]  DifferentiatorOutMax=[]  FilterDiffOutCoefMin=[]  FilterDiffOutCoefMax=[]  ReciprocalOutMin=[]  ReciprocalOutMax=[]  SumDenOutMin=[]  SumDenOutMax=[]  SumNumOutMin=[]  SumNumOutMax=[]  DivideOutMin=[]  DivideOutMax=[]  UdiffTsProdOutMin=[]  UdiffTsProdOutMax=[]  NTsProdOutMin=[]  NTsProdOutMax=[]  UintegralTsProdOutMin=[]  UintegralTsProdOutMax=[]  UngainTsProdOutMin=[]  UngainTsProdOutMax=[]  ClampingZeroOutDataTypeStr=Inherit: Inherit via back propagation  ClampingZeroOutMin=[]  ClampingZeroOutMax=[]  FilterDenConstantOutDataTypeStr=Inherit: Inherit via back propagation  FilterDenConstantOutMin=[]  FilterDenConstantOutMax=[]  PCopyOutDataTypeStr=Inherit: Inherit via back propagation  PCopyOutMin=[]  PCopyOutMax=[]  NCopyOutDataTypeStr=Inherit: Inherit via back propagation  NCopyOutMin=[]  NCopyOutMax=[]  IntegratorContinuousStateAttributes=''  IntegratorStateMustResolveToSignalObject=off  IntegratorRTWStateStorageClass=Auto  FilterContinuousStateAttributes=''  FilterStateMustResolveToSignalObject=off  FilterRTWStateStorageClass=Auto  ParallelPVariant=InternalParameters  IdealPVariant=Disabled  IVariant=InternalParameters  DVariant=Disabled  IntegratorVariant=Discrete  SatVariant=Enabled  AWVariant=Passthrough  PCopyVariant=Disabled  TRVariant=Disabled  FdbkBlocksVariant=Forward  IdealPFdbkVariant=Disabled  SatFdbkVariant=Disabled  DerivativeFilterVariant=Disabled  NVariant=Disabled  NCopyVariant=Disabled_SignalSpec  FilterICVariant=Disabled  IntegratorICVariant=InternalICs  ExternalResetVariant=Disabled  TRSumVariant=Passthrough  SumFdbkVariant=Disabled  SumVariant=Sum_PI  TsampFilterVariant=InternalTs  TsampNgainVariant=Passthrough  TsampIntegralVariant=Disabled_SignalSpec  ExternalSaturationOutDataTypeStr=Inherit: Same as second input  DerivativeSourceVariant=Disabled  PreIntVariant=InternalPreInt
  Saturation : Saturate  UpperLimit=1  LowerLimit=-1
  Scope : Scope  NumInputPorts=2
  Scope4 : Scope  NumInputPorts=2
  Sum : Sum  Inputs=|-+
  Sum1 : Sum  Inputs=|+-
  Sum2 : Sum  Inputs=|+-
  Sum3 : Sum  Inputs=|+-
  Sum{4..6,8} (4 alike) : Sum  Inputs=|++
  Switch : Switch  Criteria=u2 > Threshold  Threshold=10
  Terminator : Terminator
  Terminator1 : Terminator
  abc to dq0 : spsabctodq0Lib/abc to dq0  Alignment=90 degrees behind phase A axis
  abc to dq1 : spsabctodq0Lib/abc to dq0  Alignment=90 degrees behind phase A axis
  dq0 to abc : spsdq0toabcLib/dq0 to abc  Alignment=90 degrees behind phase A axis
  wL : Gain  Gain=0.314*0.003
  wL1 : Gain  Gain=0.314*0.003
  Pulses : Outport
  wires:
  abc to dq0/1 -> Demux/1
  Demux/3 -> Terminator/1
  Demux1/3 -> Terminator1/1
  abc to dq1/1 -> Demux1/1
  Iabc_B3/1 -> abc to dq1/1
  Constant/1 -> Sum/1
  Demux/2 -> [Vq]  "Vq"
  Sum/1 -> PID Controller/1
  PID Controller/1 -> Sum8/1
  [wt] -> abc to dq1/2, abc to dq0/2
  Demux1/1 -> [Id]  "Id"
  Demux1/2 -> [Iq]  "Iq"
  [Id] -> Scope/2, Sum1/2
  Iqref/1 -> Scope4/1, Sum2/1
  [Iq] -> Sum2/2, Scope4/2
  Sum1/1 -> PID Controller1/1
  Sum2/1 -> PID Controller2/1
  PID Controller1/1 -> Sum3/1
  PID Controller2/1 -> Sum4/1
  wL1/1 -> Sum4/2
  wL/1 -> Sum3/2
  Sum3/1 -> Sum5/1
  [Vd] -> Sum5/2
  Sum4/1 -> Sum6/1
  [Vq] -> Sum6/2
  Mux/1 -> dq0 to abc/1
  Sum5/1 -> Mux/1  "ud"
  Sum6/1 -> Mux/2  "uq"
  Constant1/1 -> Mux/3
  dq0 to abc/1 -> Gain/1
  Vabc_B3/1 -> abc to dq0/1
  Idref/1 -> Scope/1, Sum1/1
  [Id] -> wL1/1
  [Iq] -> wL/1
  Demux/1 -> [Vd]  "Vd"
  Gain/1 -> Saturation/1
  Memory/1 -> Pulses/1
  Discrete-Time Integrator/1 -> [wt]
  Saturation/1 -> Memory/1
  Constant3/1 -> Sum8/2
  Switch/1 -> Sum/2
  Constant4/1 -> Switch/3
  Clock/1 -> Switch/2
  [Vq] -> Switch/1
  [wt] -> dq0 to abc/2
  Sum8/1 -> Discrete-Time Integrator/1

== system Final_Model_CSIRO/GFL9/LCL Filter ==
  Cf : spsSeriesRLCBranchLib/Series RLC Branch  LConnTagsString=__new0  RConnTagsString=__new0  BranchType=RC  Resistance=200  Inductance=0.0058  SetiL0=off  InitialCurrent=0  Capacitance=50e-6  Setx0=off  InitialVoltage=0  Measurements=None
  Cf1 : spsSeriesRLCBranchLib/Series RLC Branch  LConnTagsString=__new0  RConnTagsString=__new0  BranchType=RC  Resistance=200  Inductance=0.0058  SetiL0=off  InitialCurrent=0  Capacitance=50e-6  Setx0=off  InitialVoltage=0  Measurements=None
  Cf2 : spsSeriesRLCBranchLib/Series RLC Branch  LConnTagsString=__new0  RConnTagsString=__new0  BranchType=RC  Resistance=200  Inductance=0.0058  SetiL0=off  InitialCurrent=0  Capacitance=50e-6  Setx0=off  InitialVoltage=0  Measurements=None
  Ground : spsGroundLib/Ground  LConnTagsString=a
  Lg : spsSeriesRLCBranchLib/Series RLC Branch  LConnTagsString=__new0  RConnTagsString=__new0  BranchType=L  Resistance=0.2  Inductance=5e-6  SetiL0=off  InitialCurrent=0  Capacitance=1e-6  Setx0=off  InitialVoltage=0  Measurements=None
  Linv : spsSeriesRLCBranchLib/Series RLC Branch  LConnTagsString=__new0  RConnTagsString=__new0  BranchType=RL  Resistance=1e-3  Inductance=0.003e-3  SetiL0=off  InitialCurrent=0  Capacitance=1e-6  Setx0=off  InitialVoltage=0  Measurements=None
  Series RLC Branch1 : spsSeriesRLCBranchLib/Series RLC Branch  LConnTagsString=__new0  RConnTagsString=__new0  BranchType=RL  Resistance=1e-3  Inductance=0.003e-3  SetiL0=off  InitialCurrent=0  Capacitance=1e-6  Setx0=off  InitialVoltage=0  Measurements=None
  Series RLC Branch2 : spsSeriesRLCBranchLib/Series RLC Branch  LConnTagsString=__new0  RConnTagsString=__new0  BranchType=RL  Resistance=1e-3  Inductance=0.003e-3  SetiL0=off  InitialCurrent=0  Capacitance=1e-6  Setx0=off  InitialVoltage=0  Measurements=None
  Series RLC Branch3 : spsSeriesRLCBranchLib/Series RLC Branch  LConnTagsString=__new0  RConnTagsString=__new0  BranchType=L  Resistance=0.2  Inductance=5e-6  SetiL0=off  InitialCurrent=0  Capacitance=1e-6  Setx0=off  InitialVoltage=0  Measurements=None
  Series RLC Branch4 : spsSeriesRLCBranchLib/Series RLC Branch  LConnTagsString=__new0  RConnTagsString=__new0  BranchType=L  Resistance=0.2  Inductance=5e-6  SetiL0=off  InitialCurrent=0  Capacitance=1e-6  Setx0=off  InitialVoltage=0  Measurements=None
  Three-Phase V-I Measurement : spsThreePhaseVIMeasurementLib/Three-Phase V-I Measurement  VoltageMeasurement=phase-to-phase  SetLabelV=on  LabelV=Vabc_B2_11  Vpu=off  VpuLL=off  CurrentMeasurement=no  SetLabelI=off  LabelI=Iabc  Ipu=off  Pbase=100e6  Vbase=500e3  OutputType=Complex  PhasorSimulation=off  PSBequivalent=0
  A : PMIOPort  Side=Left
  a : PMIOPort  Port=2  Side=Right
  B : PMIOPort  Port=3  Side=Left
  b : PMIOPort  Port=4  Side=Right
  C : PMIOPort  Port=5  Side=Left
  c : PMIOPort  Port=6  Side=Right
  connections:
  A/RConn1 -- Linv/LConn1
  B/RConn1 -- Series RLC Branch1/LConn1
  C/RConn1 -- Series RLC Branch2/LConn1
  Lg/LConn1 -- Three-Phase V-I Measurement/LConn1 -- Linv/RConn1
  Series RLC Branch4/LConn1 -- Three-Phase V-I Measurement/LConn3 -- Series RLC Branch2/RConn1
  Series RLC Branch3/LConn1 -- Three-Phase V-I Measurement/LConn2 -- Series RLC Branch1/RConn1
  Cf1/LConn1 -- Ground/LConn1 -- Cf/LConn1 -- Cf2/LConn1
  Cf/RConn1 -- Three-Phase V-I Measurement/RConn1
  Cf1/RConn1 -- Three-Phase V-I Measurement/RConn2
  Cf2/RConn1 -- Three-Phase V-I Measurement/RConn3
  Lg/RConn1 -- a/RConn1
  Series RLC Branch3/RConn1 -- b/RConn1
  Series RLC Branch4/RConn1 -- c/RConn1

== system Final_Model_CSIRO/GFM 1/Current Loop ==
  i_s_ref_dq0 : Inport
  v_dq0 : Inport  Port=2
  i_s_dq0 : Inport  Port=3
  w : Inport  Port=4
  Demux : Demux  Outputs=2
  Demux1 : Demux  Outputs=2
  Demux2 : Demux  Outputs=2
  First-Order Filter2 : spsFirstOrderFilterLib/First-Order Filter  Commented=on  FilterType=Lowpass  Tc=25e-3  Ts=0  Initialize=on  Vac_Init=[0, 0, 50]  Vdc_Init=1  PlotResponse=off  FreqRange="[0,  200,  1]"
  First-Order Filter3 : spsFirstOrderFilterLib/First-Order Filter  Commented=on  FilterType=Lowpass  Tc=25e-3  Ts=0  Initialize=on  Vac_Init=[0, 0, 50]  Vdc_Init=0  PlotResponse=off  FreqRange="[0,  200,  1]"
  Gain Corrector : Gain  Gain=Kp_i
  Gain Corrector1 : Gain  Gain=Kp_i
  Integration Time : Gain  Gain=Ki_i / Kp_i
  Integration Time 1 : Gain  Gain=Ki_i / Kp_i
  Integration Time1 : Gain  Gain=1/n
  Integration Time2 : Gain  Gain=1/n
  Integrator : Integrator  InitialCondition=0.0001
  Integrator 1 : Integrator
  Mux : Mux  Inputs=3
  Product : Product  RndMeth=Zero
  Product1 : Product  RndMeth=Zero
  Selector1 : Selector  InputPortWidth=3  IndexOptions=Index vector (dialog)  Indices=[1 2]  OutputSizes=1
  Selector2 : Selector  InputPortWidth=3  IndexOptions=Index vector (dialog)  Indices=[1 2]  OutputSizes=1
  Selector3 : Selector  InputPortWidth=3  IndexOptions=Index vector (dialog)  Indices=[1 2]  OutputSizes=1
  Sum : Sum  Inputs=|+-
  Sum1 : Sum  Inputs=|++
  Sum2 : Sum  Inputs=|+-
  Sum3 : Sum  Inputs=|++
  Sum4 : Sum  Inputs=|++
  Sum5 : Sum  Inputs=++|
  Sum6 : Sum  Inputs=-+|
  Sum7 : Sum  Inputs=++|
  Vm_0* : Constant  Value=0
  Voltage Compensator 1 : Gain  Gain=Kff_v
  Voltage compensator : Gain  Gain=Kff_v
  w*Lf_pu : Gain  Gain=L_f
  v_s_ref_dq0 : Outport  VectorParamsAs1DForOutWhenUnconnected=off
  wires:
  Sum/1 -> Integration Time/1, Integration Time1/1
  Integration Time 1/1 -> Integrator 1/1
  Integration Time/1 -> Integrator/1
  Sum5/1 -> Sum7/2
  Sum6/1 -> Integration Time 1/1, Integration Time2/1
  Demux/1 -> Sum/1
  Sum3/1 -> Mux/1  "Vm_d*"
  Sum7/1 -> Mux/2  "Vm_q*"
  Demux2/2 -> Voltage Compensator 1/1
  Voltage Compensator 1/1 -> Sum7/1
  Product/1 -> Sum2/2
  w*Lf_pu/1 -> Product1/1, Product/2
  i_s_ref_dq0/1 -> Selector1/1
  v_dq0/1 -> Selector3/1
  Integrator 1/1 -> Sum4/1
  Voltage compensator/1 -> Sum3/2
  Sum1/1 -> Gain Corrector/1
  Sum2/1 -> Sum3/1
  Sum4/1 -> Gain Corrector1/1
  Demux/2 -> Sum6/2
  Selector1/1 -> Demux/1
  Gain Corrector/1 -> Sum2/1
  w/1 -> w*Lf_pu/1
  Mux/1 -> v_s_ref_dq0/1
  Selector2/1 -> Demux1/1
  i_s_dq0/1 -> Selector2/1
  Selector3/1 -> Demux2/1
  Demux1/2 -> Product/1, Sum6/1
  Vm_0*/1 -> Mux/3
  Integrator/1 -> Sum1/1
  Demux1/1 -> Product1/2, Sum/2
  Demux2/1 -> Voltage compensator/1
  Product1/1 -> Sum5/1
  Gain Corrector1/1 -> Sum5/2
  Integration Time1/1 -> Sum1/2
  Integration Time2/1 -> Sum4/2

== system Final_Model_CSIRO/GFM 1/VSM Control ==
  p_m : Inport
  p_set : Inport  Port=2
  v_m : Inport  Port=3
  V_abc : Inport  Port=4
  w_b : Inport  Port=5
  Demux : Demux  Outputs=3
  First-Order Filter2 : spsFirstOrderFilterLib/First-Order Filter  FilterType=Lowpass  Tc=25e-3  Ts=0  Initialize=on  Vac_Init=[0, 0, 50]  Vdc_Init=1  PlotResponse=off  FreqRange="[0,  200,  1]"
  Gain17 : Gain  Gain=1/(w_b)
  Gain2 : Gain  Gain=1/(w_b)
  Gain5 : Gain  Gain=D_p
  Gain6 : Gain  Gain=1/J
  Integrator : Integrator
  Integrator2 : Integrator
  MATLAB Function1 : MATLAB Function  TreatAsAtomicUnit=on
  PID Controller : slpidlib/PID Controller  Controller=PID  Form=Parallel  TimeDomain=Continuous-time  UseExternalTs=off  SampleTime=-1  IntegratorMethod=Forward Euler  FilterMethod=Forward Euler  ControllerParametersSource=internal  P=kp_v_ac  I=ki_v_ac  UseKiTs=off  D=0  UseExternalDerivativeSource=off  N=100  UseFilter=on  TunerSelectOption=Transfer Function Based (PID Tuner App)  InitialConditionSource=internal  InitialConditionForIntegrator=0  InitialConditionForFilter=0  DifferentiatorICPrevScaledInput=0  ExternalReset=none  TrackingMode=off  Kt=1  LimitOutput=off  SatLimitsSource=internal  UpperSaturationLimit=inf  LowerSaturationLimit=-inf  LinearizeAsGain=on  AntiWindupMode=none  Kb=1  LimitIntegrator=off  UpperIntegratorSaturationLimit=inf  LowerIntegratorSaturationLimit=-inf  POutMin=[]  POutMax=[]  IOutMin=[]  IOutMax=[]  DOutMin=[]  DOutMax=[]  NOutMin=[]  NOutMax=[]  SumOutMin=[]  SumOutMax=[]  SaturationOutMin=[]  SaturationOutMax=[]  PParamMin=[]  PParamMax=[]  IParamMin=[]  IParamMax=[]  DParamMin=[]  DParamMax=[]  NParamMin=[]  NParamMax=[]  KbParamMin=[]  KbParamMax=[]  KtParamMin=[]  KtParamMax=[]  KbOutMin=[]  KbOutMax=[]  KtOutMin=[]  KtOutMax=[]  IntegratorOutMin=[]  IntegratorOutMax=[]  FilterOutMin=[]  FilterOutMax=[]  SumI1OutMin=[]  SumI1OutMax=[]  SumI2OutMin=[]  SumI2OutMax=[]  SumI3OutMin=[]  SumI3OutMax=[]  SumI4OutMin=[]  SumI4OutMax=[]  SumDOutMin=[]  SumDOutMax=[]  DifferentiatorOutMin=[]  DifferentiatorOutMax=[]  FilterDiffOutCoefMin=[]  FilterDiffOutCoefMax=[]  ReciprocalOutMin=[]  ReciprocalOutMax=[]  SumDenOutMin=[]  SumDenOutMax=[]  SumNumOutMin=[]  SumNumOutMax=[]  DivideOutMin=[]  DivideOutMax=[]  UdiffTsProdOutMin=[]  UdiffTsProdOutMax=[]  NTsProdOutMin=[]  NTsProdOutMax=[]  UintegralTsProdOutMin=[]  UintegralTsProdOutMax=[]  UngainTsProdOutMin=[]  UngainTsProdOutMax=[]  ClampingZeroOutDataTypeStr=Inherit: Inherit via back propagation  ClampingZeroOutMin=[]  ClampingZeroOutMax=[]  FilterDenConstantOutDataTypeStr=Inherit: Inherit via back propagation  FilterDenConstantOutMin=[]  FilterDenConstantOutMax=[]  PCopyOutDataTypeStr=Inherit: Inherit via back propagation  PCopyOutMin=[]  PCopyOutMax=[]  NCopyOutDataTypeStr=Inherit: Inherit via back propagation  NCopyOutMin=[]  NCopyOutMax=[]  IntegratorContinuousStateAttributes=''  IntegratorStateMustResolveToSignalObject=off  IntegratorRTWStateStorageClass=Auto  FilterContinuousStateAttributes=''  FilterStateMustResolveToSignalObject=off  FilterRTWStateStorageClass=Auto  ParallelPVariant=InternalParameters  IdealPVariant=Disabled  IVariant=InternalParameters  DVariant=InternalParameters  IntegratorVariant=Continuous  SatVariant=Disabled  AWVariant=Passthrough  PCopyVariant=Disabled  TRVariant=Disabled  FdbkBlocksVariant=Forward  IdealPFdbkVariant=Disabled  SatFdbkVariant=Disabled  DerivativeFilterVariant=ContFilter  NVariant=InternalParameters  NCopyVariant=Disabled  FilterICVariant=InternalICsFilter  IntegratorICVariant=InternalICs  ExternalResetVariant=Disabled  TRSumVariant=Passthrough  SumFdbkVariant=Disabled  SumVariant=Sum_PID  TsampFilterVariant=InternalTs  TsampNgainVariant=Passthrough  TsampIntegralVariant=Disabled_SignalSpec  ExternalSaturationOutDataTypeStr=Inherit: Same as second input  DerivativeSourceVariant=ErrorSignal  PreIntVariant=InternalPreInt
  Sum : Sum  Inputs=+|+|-
  Sum1 : Sum  Inputs=-+|
  Sum2 : Sum  Inputs=+|-
  Terminator : Terminator
  Terminator1 : Terminator
  Transfer Fcn1 : TransferFcn  Numerator=[w_f]  Denominator=[1 w_f]
  abc to dq1 : spsabctodq0Lib/abc to dq0  Alignment=90 degrees behind phase A axis
  abc to dq2 : spsabctodq0Lib/abc to dq0  Alignment=90 degrees behind phase A axis
  w_ref : Outport  VectorParamsAs1DForOutWhenUnconnected=off
  theta_ref : Outport  Port=2  VectorParamsAs1DForOutWhenUnconnected=off
  v_ref_dq0 : Outport  Port=3  VectorParamsAs1DForOutWhenUnconnected=off
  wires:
  abc to dq2/1 -> v_ref_dq0/1
  MATLAB Function1/1(e) -> abc to dq2/1
  PID Controller/1 -> MATLAB Function1/1(M_fi_f)
  p_set/1 -> Gain2/1
  Gain5/1 -> Sum/1
  Gain17/1 -> Sum/3
  Gain6/1 -> Integrator/1
  Gain2/1 -> Sum/2
  Sum2/1 -> Gain5/1
  Integrator2/1 -> theta_ref/1, abc to dq2/2, MATLAB Function1/2(theta), abc to dq1/2
  Transfer Fcn1/1 -> Gain17/1
  Integrator/1 -> MATLAB Function1/3(w), w_ref/1, Sum2/2, Integrator2/1
  w_b/1 -> Sum2/1
  Demux/3 -> Terminator1/1
  Demux/2 -> Terminator/1
  Demux/1 -> Sum1/1
  V_abc/1 -> abc to dq1/1
  abc to dq1/1 -> Demux/1
  Sum1/1 -> PID Controller/1
  v_m/1 -> Sum1/2
  Sum/1 -> Gain6/1
  p_m/1 -> First-Order Filter2/1
  First-Order Filter2/1 -> Transfer Fcn1/1

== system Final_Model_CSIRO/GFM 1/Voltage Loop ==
  v_ref_dq0 : Inport
  v_dq0 : Inport  Port=2
  i_dq0 : Inport  Port=3
  w : Inport  Port=4
  Current Compensator : Gain  Gain=Kff_i
  Current Compensator1 : Gain  Gain=Kff_i
  Damping (d) : Gain  Gain=Kp_v
  Damping (q) : Gain  Gain=Kp_v
  Demux : Demux  Outputs=2
  Demux1 : Demux  Outputs=2
  Demux2 : Demux  Outputs=2
  Eg_d * (wCf) : Product  RndMeth=Zero
  "Eg_q * (wCf) " : Product  RndMeth=Zero
  Filter capacitance : Gain  Gain=C_f
  Integration Time : Gain  Gain=Ki_v / Kp_v
  Integration Time1 : Gain  Gain=Ki_v / Kp_v
  Integration Time2 : Gain  Gain=n
  Integration Time3 : Gain  Gain=n
  Integrator : Integrator
  Integrator1 : Integrator
  Is_0* : Constant  Value=0
  Mux : Mux  Inputs=3
  Selector : Selector  InputPortWidth=3  IndexOptions=Index vector (dialog)  Indices=[1 2]  OutputSizes=1
  Selector1 : Selector  InputPortWidth=3  IndexOptions=Index vector (dialog)  Indices=[1 2]  OutputSizes=1
  Selector2 : Selector  InputPortWidth=3  IndexOptions=Index vector (dialog)  Indices=[1 2]  OutputSizes=1
  Sum : Sum  Inputs=|+-
  Sum1 : Sum  Inputs=|++
  Sum2 : Sum  Inputs=|+-
  Sum3 : Sum  Inputs=|++
  Sum4 : Sum  Inputs=|++
  Sum5 : Sum  Inputs=++|
  Sum6 : Sum  Inputs=-+|
  Sum7 : Sum  Inputs=++|
  i_s_ref_dq0 : Outport  VectorParamsAs1DForOutWhenUnconnected=off
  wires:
  Is_0*/1 -> Mux/3
  w/1 -> Filter capacitance/1
  Integration Time1/1 -> Integrator1/1
  Integrator1/1 -> Sum4/1
  Demux/2 -> Sum6/2  "Eg_q*"
  v_ref_dq0/1 -> Selector1/1
  Eg_d * (wCf)/1 -> Sum5/1  "Is_f"
  Sum7/1 -> Mux/2  "Is_q*"
  Demux2/2 -> Current Compensator1/1  "Ig_q"
  Demux/1 -> Sum/1  "Eg_d*"
  Sum6/1 -> Integration Time3/1, Integration Time1/1
  Demux2/1 -> Current Compensator/1  "Ig_d"
  Sum2/1 -> Sum3/1  "Is_d'"
  Current Compensator/1 -> Sum3/2
  Demux1/1 -> Eg_d * (wCf)/1, Sum/2  "Eg_d"
  Current Compensator1/1 -> Sum7/1
  "Eg_q * (wCf) "/1 -> Sum2/2  "Is_f"
  Demux1/2 -> "Eg_q * (wCf) "/1, Sum6/1  "Eg_q"
  Filter capacitance/1 -> "Eg_q * (wCf) "/2, Eg_d * (wCf)/2
  Damping (d)/1 -> Sum2/1  "Is_d\""
  i_dq0/1 -> Selector2/1
  Sum5/1 -> Sum7/2  "Is_q'"
  Sum1/1 -> Damping (d)/1
  Integrator/1 -> Sum1/1
  Integration Time/1 -> Integrator/1
  Sum4/1 -> Damping (q)/1
  v_dq0/1 -> Selector/1
  Damping (q)/1 -> Sum5/2  "Is_q\""
  Selector/1 -> Demux1/1
  Selector1/1 -> Demux/1
  Selector2/1 -> Demux2/1
  Mux/1 -> i_s_ref_dq0/1
  Sum/1 -> Integration Time/1, Integration Time2/1
  Integration Time2/1 -> Sum1/2
  Integration Time3/1 -> Sum4/2
  Sum3/1 -> Mux/1  "Is_d*"
